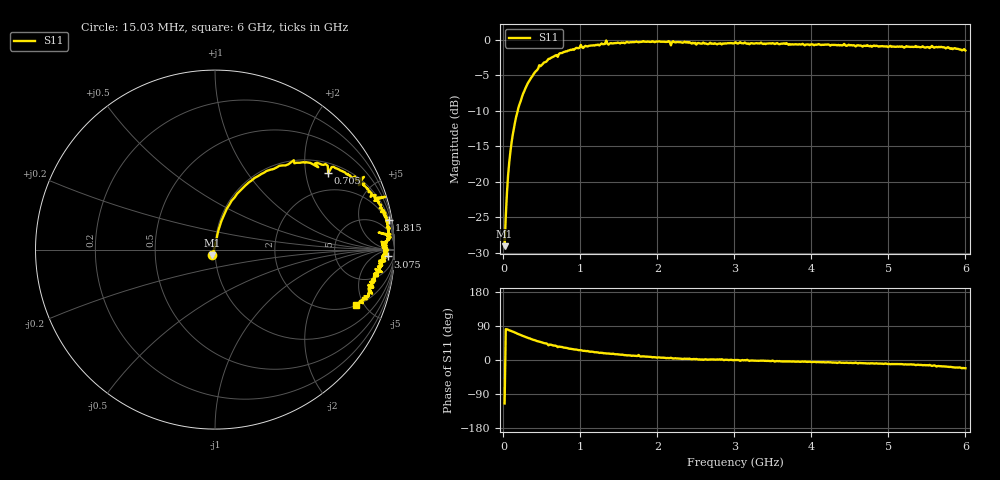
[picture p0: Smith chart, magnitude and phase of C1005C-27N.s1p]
!	Network	Analyzer	HP8753E.07.74:	Oct	30	2002	Serial	No.	JP38451487
!	Hewlett-Packard
!	7	Sep	2009	9:01:41
!	Frequency	S11
#	HZ	S	RI	R	50
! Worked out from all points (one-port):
!   400 points, 15.03 MHz to 6 GHz, reference 50 ohm
!   lowest |S11| = -29.1 dB at 15.03 MHz (marker M1), VSWR 1.07, Z = 48.5 - j3.1 ohm
!   |S11| at or under -10 dB: start of sweep to 184.6 MHz
!   S11 on the Smith chart (normalised r, x): 15.03 MHz: 0.97, -0.06; 705 MHz: 1.33, +2.68; 1.815 GHz: 1, +12; 3.075 GHz: 25, -28; 6 GHz: 2.01, -4.34
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1.502992e7  -0.0147 -0.032
4.502978e7  0.013 0.0818
7.502962e7  0.0277 0.134
1.200294e8  0.056 0.206
1.95029e8  0.123 0.311
4.650277e8  0.439 0.498
7.050265e8  0.631 0.425
7.650262e8  0.672 0.454
1.005025e9  0.83 0.405
1.320023e9  0.894 0.288
1.335023e9  0.948 0.294
1.365023e9  0.887 0.272
1.515022e9  0.917 0.23
1.740021e9  0.953 0.177
1.755021e9  0.938 0.221
1.815021e9  0.968 0.164
2.145019e9  0.978 0.0852
2.175019e9  0.912 0.0952
2.205019e9  0.979 0.0684
2.265019e9  0.967 0.0688
3.015015e9  0.964 -0.00226
3.075015e9  0.964 -0.038
3.165014e9  0.94 0.00858
3.195014e9  0.932 -0.0395
3.765011e9  0.928 -0.062
4.515007e9  0.913 -0.119
5.265004e9  0.878 -0.183
6e9  0.784 -0.311
